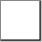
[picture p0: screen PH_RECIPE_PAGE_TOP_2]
VISUALIZATION PH_RECIPE_PAGE_TOP_2  // 42x42
VAR_IN_OUT
	RECIPE_CTRL_V2 : None;
END_VAR
    Rectangle (0,0 40x40)
        tap RECIPE_CTRL_V2.sCmd.bJumpTop
    Polyline (35,10), colour toggle: (RECIPE_CTRL_V2.sCmd.bJumpTop) <> 0
        tap RECIPE_CTRL_V2.sCmd.bJumpTop
    Polygon (20,20), colour toggle: (RECIPE_CTRL_V2.sCmd.bJumpTop) <> 0
        tap RECIPE_CTRL_V2.sCmd.bJumpTop
    Polygon (20,10), colour toggle: (RECIPE_CTRL_V2.sCmd.bJumpTop) <> 0
        tap RECIPE_CTRL_V2.sCmd.bJumpTop
END_VISUALIZATION
